FUNCTION_BLOCK IC_KP2_2HB21_IQH3_SF
VAR_INPUT
	pADR_IN:								PVOID;					(* Pointer array input data *)
	cbSIZE_IN:								UDINT;					(* Size array input data *)
	pADR_OUT:								PVOID;					(* Pointer array output data *)
	cbSIZE_OUT:								UDINT;					(* Size array output data *)	
	I_T_Timeout : 							TIME;					// Timeout to check command responses
	I_b_StartRead : 						BOOL;					// Trigger to start read command
	I_b_StartWrite : 						BOOL;					// Trigger to start write command
	I_b_StartSpecialCommand : 				BOOL;					// Trigger to start special command (user defined command)
	I_b_UserMemory_UID : 					BOOL;					//0 := access to User Memory; 1 := access to UID/Fixcode
	I_b_EPC : 								BOOL;					//0 := configuration done by Head1UserMemoryUID active; 1 := access to UII/EPC Code (UHF only)
	I_b_SingleEnhanced : 					BOOL;					// 0 = Single command (one-time) ; 1 = Enhanced command (permanent)
	I_b_Quit : 								BOOL;					// Trigger to start Quit command (abort Enhanced command)
	I_w_StartAddress : 						WORD;					// Startaddress of memory access 
	I_i_WordNumber : 						INT;					// Number of blocks
	I_w_TagType : 							WORD;					// TagType
	I_b_WriteParameter : 					BOOL;					//0 := read access to parameter; 1 := write access to parameter
END_VAR
VAR_OUTPUT
	O_b_Done : 								BOOL;					//0 = tag leave detection zone (Enhanced); 1 = tag access successfully executed
	O_b_NoDataCarrier : 					BOOL;					//0 = tag inside/enter detection zone; 1 = no tag or tag leave detection zone
	O_b_Busy : 								BOOL;					//0 = no command actiive; 1 = command active
	O_b_Finish : 							BOOL;					//0 = command active; 1 = command finished
	O_b_Error : 							BOOL;					//0 = no error state; 1 = error state active; check status value
	O_B_Status : 							BYTE;					//Status value of the command response; error information
	O_B_ReplyCounter : 						BYTE;					//Counter of the command responses; increment each new response
	O_b_EndConfig : 						BOOL;					//1 = parameter access finished
END_VAR
VAR_IN_OUT
	IO_b_SetRestart : 						BOOL;					//Trigger initialisation routine
	IO_b_InitFinish : 						BOOL;					//Initialisation routine finished
	IO_b_StartConfig : 						BOOL;
	UserDataGlobal 	: 						IDENTControl_UserData;	//Data block for read/write data and parameter data
END_VAR
VAR
	IDENTControl_FB_SF		: 				IDENTControl_SF;		//Definition of internal function block for Single Frame Protocol
	SpecialCommand_Internal: 				BOOL;					//internal signal for trigger of Special command
	ConfigActive : 							BOOL;					//execution of Special command active
	StateConfig : 							INT;					//state of the execution list
	Done_Internal : 						BOOL;					//Special command finished
	i : 									INT := 0;				//counter
END_VAR

	(*
	#############################################################################################
	
	General Header
	------------------------------------------------------------------------------------------
	Short description:  Function Block for IC-KP2-2HB21 SingleFrame with Parameter configuration for IQH3-FP-V1
	Version:            1.0
	Name:               IC-KP2-2HB21 Singleframe Protocol with HF Parameter configuration for IQH3-FP-V1
	Date:               2024-10-08
	Company:            Pepperl+Fuchs SE
	Author:             Karsten Reinhardt
	EMail:              kreinhardt@de.pepperl-fuchs.com
	Phone:              +49 (0) 621 776 1736

	Changes 1.0: first release
	    - function block include a further function block for standard read/write command without automatic parameter
	    configuration;    
	    - read and write access for different HF parameter
		- based on function block for IC-KP2-1HB17 TIA Portal Profinet for parameter access of IQH3-FP-V1
	
	------------------------------------------------------------------------------------------
	    
	#############################################################################################
	*)

	(*input SpecialCommand hand over to internal signal*)
	SpecialCommand_Internal                   			:= I_b_StartSpecialCommand;

	(*Increase the state of the configuration counter*)
	IF ConfigActive = TRUE AND O_b_Done = TRUE THEN
	    ConfigActive                         			:= FALSE;
	    StateConfig                          			:= StateConfig + 1;
	END_IF;
	
	(*Set Status of the configuration counter to 1 with the trigger for the start of the configuration*)
	IF IO_b_StartConfig = TRUE THEN
	    StateConfig                          			:= 1;
	    IO_b_StartConfig                          		:= FALSE;
	    O_b_EndConfig                             		:= FALSE;
	END_IF;

	IF NOT ConfigActive THEN
	    CASE StateConfig OF
	            
	        0: (* ***** Idle state ***** *)
	            ;
	            
	        1:  (*Additional Information - Parameter IF; transmit a further information telegram with RSSI value;
	            if this parameter is activated a further status 16#0B telegram will transmitted by the evaluation
	            unit; this telegram follows directly after the status 16#00 telegram which contains the read in data
	            of a tag; the status 16#0B telegram with the information will send only one time after the tag is detected;
	            in default setting the parameter is switched off and no additional information are transmit*)
	            IF I_b_WriteParameter = TRUE THEN
	                UserDataGlobal.SpecialCommand[0] 	:= 16#BF;
	            ELSE
					UserDataGlobal.SpecialCommand[0] 	:= 16#BE;	                
	            END_IF;
	            UserDataGlobal.SpecialCommand[1]        := 16#00;
	            UserDataGlobal.SpecialCommand[2]        := 16#00;
	            UserDataGlobal.SpecialCommand[3]        := 16#51;      //SystemCode Q
	            UserDataGlobal.SpecialCommand[4]        := 16#49;      //Parameter sign High Byte 'I'
	            UserDataGlobal.SpecialCommand[5]        := 16#46;      //Parameter sign Low Byte 'F'
				IF I_b_WriteParameter = TRUE THEN
	                UserDataGlobal.SpecialCommand[6]    := 16#00;    //Length Parameter High Byte 
	                UserDataGlobal.SpecialCommand[7]    := 16#01;    //Length Parameter Low Byte 
	                UserDataGlobal.SpecialCommand[8]    := UserDataGlobal.WriteParam_IF;    //Parameter value; 16#00 Switched off; 16#01 Switched on
	            ELSE
	                UserDataGlobal.SpecialCommand[6]    := 16#00;    //Length Parameter High Byte 
	                UserDataGlobal.SpecialCommand[7]    := 16#00;    //Length Parameter Low Byte 
	                UserDataGlobal.SpecialCommand[8]    := 16#00;
	            END_IF;
	            SpecialCommand_Internal       			:= TRUE;
	            ConfigActive                 			:= TRUE;            
				
	        2:  (*AFI to request - Parameter AF; *)
	            IF I_b_WriteParameter = TRUE THEN
	                UserDataGlobal.SpecialCommand[0]    := 16#BF;
	            ELSE
	                UserDataGlobal.SpecialCommand[0]    := 16#BE;
	            END_IF;
	            UserDataGlobal.SpecialCommand[1]        := 16#00;
	            UserDataGlobal.SpecialCommand[2]        := 16#00;
	            UserDataGlobal.SpecialCommand[3]        := 16#51;      //SystemCode Q
	            UserDataGlobal.SpecialCommand[4]        := 16#41;      //Parameter sign High Byte 'A'
	            UserDataGlobal.SpecialCommand[5]        := 16#46;      //Parameter sign Low Byte 'F'
	            IF I_b_WriteParameter = TRUE THEN
	                UserDataGlobal.SpecialCommand[6]    := 16#00;    //Length Parameter High Byte 
	                UserDataGlobal.SpecialCommand[7]    := 16#01;    //Length Parameter Low Byte 
	                UserDataGlobal.SpecialCommand[8]    := UserDataGlobal.WriteParam_AF;    //Parameter value; 16#00 = all tags; Range between 16#00 and 16#FF
	            ELSE
	                UserDataGlobal.SpecialCommand[6]    := 16#00;    //Length Parameter High Byte 
	                UserDataGlobal.SpecialCommand[7]    := 16#00;    //Length Parameter Low Byte 
	                UserDataGlobal.SpecialCommand[8]    := 16#00;    //Parameter value; 
	            END_IF;
	            SpecialCommand_Internal       			:= TRUE;
	            ConfigActive 							:= TRUE;

	        3:  (*Enhanced Status 5 - Parameter E5; delay the sending of a status 16#05 telegram which signalise that
	            a tag leaves the detection zone; if there is a inhomogeneous reading zone you have areas in which a tag
	            could not identified; in this case the reader generates a status 16#05 telegram that signalize that a tag 
	            could not accessed; these parameter can delay such telegrams that you can avoid a lot of status 16#05 (no read) 
	            telegrams in a inhomogeneous reading zone*)
	            IF I_b_WriteParameter = TRUE THEN
	                UserDataGlobal.SpecialCommand[0]    := 16#BF;
	            ELSE
	                UserDataGlobal.SpecialCommand[0]    := 16#BE;
	            END_IF;
	            UserDataGlobal.SpecialCommand[1]        := 16#00;
	            UserDataGlobal.SpecialCommand[2]        := 16#00;
	            UserDataGlobal.SpecialCommand[3]        := 16#51;      //SystemCode Q
	            UserDataGlobal.SpecialCommand[4]        := 16#45;      //Parameter sign High Byte 'E'
	            UserDataGlobal.SpecialCommand[5]        := 16#35;      //Parameter sign Low Byte '5'
	            IF I_b_WriteParameter = TRUE THEN
	                UserDataGlobal.SpecialCommand[6]    := 16#00;    //Length Parameter High Byte 
	                UserDataGlobal.SpecialCommand[7]    := 16#01;    //Length Parameter Low Byte 
	                UserDataGlobal.SpecialCommand[8]    := UserDataGlobal.WriteParam_E5;    //Parameter value; value Parameter E5
	                UserDataGlobal.SpecialCommand[9]    := 16#00;    //Parameter value; 
	                UserDataGlobal.SpecialCommand[10]   := 16#00;    //Parameter value; 
	                UserDataGlobal.SpecialCommand[11]   := 16#00;    //Parameter value; 
	            ELSE
	                UserDataGlobal.SpecialCommand[6]    := 16#00;    //Length Parameter High Byte 
	                UserDataGlobal.SpecialCommand[7]    := 16#00;    //Length Parameter Low Byte 
	                UserDataGlobal.SpecialCommand[8]    := 16#00;    //Parameter value; 
	                UserDataGlobal.SpecialCommand[9]    := 16#00;    //Parameter value; 
	                UserDataGlobal.SpecialCommand[10]   := 16#00;    //Parameter value; 
	                UserDataGlobal.SpecialCommand[11]   := 16#00;    //Parameter value; 
	            END_IF;
	            SpecialCommand_Internal       			:= TRUE;
	            ConfigActive                 			:= TRUE;

 			4:  (*Number of Tags - Parameter NT; stop criteria to abort the execution of a Single command; this parameter
	            allows the stop of the command execution if one or a defined number of tags are detected; in default setting
	            the parameter has the value 16#FF and the command does not stop before all invetury rounds are executed; if
	            the value 16#01 is defined the command execution of a Single command stops if one tag is detected during an
	            invetury round; if two tags are detected during an inventury round both tags will transmit*)
	            IF I_b_WriteParameter = TRUE THEN
	                UserDataGlobal.SpecialCommand[0]    := 16#BF;
	            ELSE
	                UserDataGlobal.SpecialCommand[0]    := 16#BE;
	            END_IF;
	            UserDataGlobal.SpecialCommand[1]        := 16#00;
	            UserDataGlobal.SpecialCommand[2]        := 16#00;
	            UserDataGlobal.SpecialCommand[3]        := 16#51;      //SystemCode Q
	            UserDataGlobal.SpecialCommand[4]        := 16#4E;      //Parameter sign High Byte 'N'
	            UserDataGlobal.SpecialCommand[5]        := 16#54;      //Parameter sign Low Byte 'T'
	            IF I_b_WriteParameter = TRUE THEN
	                UserDataGlobal.SpecialCommand[6]    := 16#00;    //Length Parameter High Byte 
	                UserDataGlobal.SpecialCommand[7]    := 16#01;    //Length Parameter Low Byte 
	                UserDataGlobal.SpecialCommand[8]    := UserDataGlobal.WriteParam_NT;    //Parameter value; 16#FF = Switched off; Default setting
	            ELSE
	                UserDataGlobal.SpecialCommand[6]    := 16#00;    //Length Parameter High Byte 
	                UserDataGlobal.SpecialCommand[7]    := 16#00;    //Length Parameter Low Byte 
	                UserDataGlobal.SpecialCommand[8]    := 16#00;    //Parameter value;
	            END_IF;
	            SpecialCommand_Internal       			:= TRUE;
	            ConfigActive                 			:= TRUE;

	        5: (*Protocol Mode - Parameter QV; defines the communication protocol of the head; in default setting the
	            head communicates with the SingleFrame protocol; this allows the identification of several tags inside
	            the detection zone; it is possible to switch the protocol to MultiFrame, but than the function block
	            is incompatible*)
	            IF I_b_WriteParameter = TRUE THEN
	                UserDataGlobal.SpecialCommand[0]    := 16#BF;
	            ELSE
	                UserDataGlobal.SpecialCommand[0]    := 16#BE;
	            END_IF;
	            UserDataGlobal.SpecialCommand[1]        := 16#00;
	            UserDataGlobal.SpecialCommand[2]        := 16#00;
	            UserDataGlobal.SpecialCommand[3]        := 16#51;      //SystemCode Q
	            UserDataGlobal.SpecialCommand[4]        := 16#51;      //Parameter sign High Byte 'Q'
	            UserDataGlobal.SpecialCommand[5]        := 16#56;      //Parameter sign Low Byte 'V'
	            IF I_b_WriteParameter = TRUE THEN
	                UserDataGlobal.SpecialCommand[6]    := 16#00;    //Length Parameter High Byte 
	                UserDataGlobal.SpecialCommand[7]    := 16#01;    //Length Parameter Low Byte 
	                UserDataGlobal.SpecialCommand[8]    := UserDataGlobal.WriteParam_QV;    //Parameter value; 
	            ELSE
	                UserDataGlobal.SpecialCommand[6]    := 16#00;    //Length Parameter High Byte 
	                UserDataGlobal.SpecialCommand[7]    := 16#00;    //Length Parameter Low Byte 
	                UserDataGlobal.SpecialCommand[8]    := 16#00;    //Parameter value; 
	            END_IF;
	            SpecialCommand_Internal       			:= TRUE;
	            ConfigActive                 			:= TRUE;
	            
	        6:  (*Q Value - Parameter QW; defines the number of time slots on the air interface with 2^Q; the number of
	            time slots should be fit to the number of tags which should be identified*)
	            IF I_b_WriteParameter = TRUE THEN
	                UserDataGlobal.SpecialCommand[0]    := 16#BF;
	            ELSE
	                UserDataGlobal.SpecialCommand[0]    := 16#BE;
	            END_IF;
	            UserDataGlobal.SpecialCommand[1]        := 16#00;
	            UserDataGlobal.SpecialCommand[2]        := 16#00;
	            UserDataGlobal.SpecialCommand[3]        := 16#51;      //SystemCode Q
	            UserDataGlobal.SpecialCommand[4]        := 16#51;      //Parameter sign High Byte 'Q'
	            UserDataGlobal.SpecialCommand[5]        := 16#57;      //Parameter sign Low Byte 'W'
	            IF I_b_WriteParameter = TRUE THEN
	                UserDataGlobal.SpecialCommand[6]    := 16#00;    //Length Parameter High Byte 
	                UserDataGlobal.SpecialCommand[7]    := 16#01;    //Length Parameter Low Byte 
	                UserDataGlobal.SpecialCommand[8]    := UserDataGlobal.WriteParam_QW;    //Parameter value; 
	            ELSE
	                UserDataGlobal.SpecialCommand[6]    := 16#00;    //Length Parameter High Byte 
	                UserDataGlobal.SpecialCommand[7]    := 16#00;    //Length Parameter Low Byte 
	                UserDataGlobal.SpecialCommand[8]    := 16#00;    //Parameter value; 
	            END_IF;
	            SpecialCommand_Internal       			:= TRUE;
	            ConfigActive                 			:= TRUE;
	            
	        7:  (*Tries allowed - Parameter TA; defines the number of allowed tries for the identification of a tag*)
	            IF I_b_WriteParameter = TRUE THEN
	                UserDataGlobal.SpecialCommand[0]    := 16#BF;
	            ELSE
	                UserDataGlobal.SpecialCommand[0]    := 16#BE;
	            END_IF;
	            UserDataGlobal.SpecialCommand[1]        := 16#00;
	            UserDataGlobal.SpecialCommand[2]        := 16#00;
	            UserDataGlobal.SpecialCommand[3]        := 16#51;      //SystemCode Q
	            UserDataGlobal.SpecialCommand[4]        := 16#54;      //Parameter sign High Byte 'T'
	            UserDataGlobal.SpecialCommand[5]        := 16#41;      //Parameter sign Low Byte 'A'
	            IF I_b_WriteParameter = TRUE THEN
	                UserDataGlobal.SpecialCommand[6]    := 16#00;    //Length Parameter High Byte 
	                UserDataGlobal.SpecialCommand[7]    := 16#01;    //Length Parameter Low Byte 
	                UserDataGlobal.SpecialCommand[8]    := UserDataGlobal.WriteParam_TA;    //Parameter value; 
	            ELSE
	                UserDataGlobal.SpecialCommand[6]    := 16#00;    //Length Parameter High Byte 
	                UserDataGlobal.SpecialCommand[7]    := 16#00;    //Length Parameter Low Byte 
	                UserDataGlobal.SpecialCommand[8]    := 16#00;    //Parameter value; 
	            END_IF;
	            SpecialCommand_Internal       			:= TRUE;
	            ConfigActive                 			:= TRUE;

			8:  (*Power Transmit - Parameter PT; defines the output power of the RFID antenna; value between 16#0001 up tp 16#0004
	            16#0001 = Min; 16#0002 = Eco; 16#0003 = Normal; 16#0004 = Max Power*)
	            IF I_b_WriteParameter = TRUE THEN
	                UserDataGlobal.SpecialCommand[0]    := 16#BF;
	            ELSE
	                UserDataGlobal.SpecialCommand[0]    := 16#BE;
	            END_IF;
	            UserDataGlobal.SpecialCommand[1]        := 16#00;
	            UserDataGlobal.SpecialCommand[2]        := 16#00;
	            UserDataGlobal.SpecialCommand[3]        := 16#51;      //SystemCode Q
	            UserDataGlobal.SpecialCommand[4]        := 16#50;      //Parameter sign High Byte 'P'
	            UserDataGlobal.SpecialCommand[5]        := 16#54;      //Parameter sign Low Byte 'T'
	            IF I_b_WriteParameter = TRUE THEN
	                UserDataGlobal.SpecialCommand[6]    := 16#00;    //Length Parameter High Byte 
	                UserDataGlobal.SpecialCommand[7]    := 16#02;    //Length Parameter Low Byte 
	                UserDataGlobal.SpecialCommand[8]    := WORD_TO_BYTE( SHL(UserDataGlobal.WriteParam_PT, 8));
	                UserDataGlobal.SpecialCommand[9]    := WORD_TO_BYTE(UserDataGlobal.WriteParam_PT);
	            ELSE
	                UserDataGlobal.SpecialCommand[6]    := 16#00;    //Length Parameter High Byte 
	                UserDataGlobal.SpecialCommand[7]    := 16#00;    //Length Parameter Low Byte 
	                UserDataGlobal.SpecialCommand[8]    := 16#00;    //Parameter value; 
	                UserDataGlobal.SpecialCommand[9]    := 16#00;    //Parameter value; 
	            END_IF;
	            SpecialCommand_Internal       			:= TRUE;
	            ConfigActive                 			:= TRUE;
				
			9:  (*Data Rate - Parameter DR; Data Rate for read operation; Default is 16#00 = normal; fast read mode = 16#01; valid for IQC21/33/34/37/39/50 *)
	            IF I_b_WriteParameter = TRUE THEN
	                UserDataGlobal.SpecialCommand[0]    := 16#BF;
	            ELSE
	                UserDataGlobal.SpecialCommand[0]    := 16#BE;
	            END_IF;
	            UserDataGlobal.SpecialCommand[1]        := 16#00;
	            UserDataGlobal.SpecialCommand[2]        := 16#00;
	            UserDataGlobal.SpecialCommand[3]        := 16#51;      //SystemCode Q
	            UserDataGlobal.SpecialCommand[4]        := 16#44;      //Parameter sign High Byte 'D'
	            UserDataGlobal.SpecialCommand[5]        := 16#52;      //Parameter sign Low Byte 'R'
	            IF I_b_WriteParameter = TRUE THEN
	                UserDataGlobal.SpecialCommand[6]    := 16#00;    //Length Parameter High Byte 
	                UserDataGlobal.SpecialCommand[7]    := 16#01;    //Length Parameter Low Byte 
	                UserDataGlobal.SpecialCommand[8]    := UserDataGlobal.WriteParam_DR;    //Parameter value; 
	                UserDataGlobal.SpecialCommand[9]    := 16#00;    //Parameter value; 
	            ELSE
	                UserDataGlobal.SpecialCommand[6]    := 16#00;    //Length Parameter High Byte 
	                UserDataGlobal.SpecialCommand[7]    := 16#00;    //Length Parameter Low Byte 
	                UserDataGlobal.SpecialCommand[8]    := 16#00;    //Parameter value; 
	                UserDataGlobal.SpecialCommand[9]    := 16#00;    //Parameter value; 
	            END_IF;
	            SpecialCommand_Internal       			:= TRUE;
	            ConfigActive                 			:= TRUE;
				
	        10:  (*Tag ID filterung on UID - Parameter TI; leading part of the UID*)
	            IF I_b_WriteParameter = TRUE THEN
	                UserDataGlobal.SpecialCommand[0]    := 16#BF;
	            ELSE
	                UserDataGlobal.SpecialCommand[0]    := 16#BE;
	            END_IF;
	            UserDataGlobal.SpecialCommand[1]        := 16#00;
	            UserDataGlobal.SpecialCommand[2]        := 16#00;
	            UserDataGlobal.SpecialCommand[3]        := 16#51;      //SystemCode Q
	            UserDataGlobal.SpecialCommand[4]        := 16#54;      //Parameter sign High Byte 'T'
	            UserDataGlobal.SpecialCommand[5]        := 16#49;      //Parameter sign Low Byte 'I'
	            IF I_b_WriteParameter = TRUE THEN
	                UserDataGlobal.SpecialCommand[6]    := UserDataGlobal.WriteParam_TI[0];    //Length Parameter High Byte 
	                UserDataGlobal.SpecialCommand[7]    := UserDataGlobal.WriteParam_TI[1];    //Length Parameter Low Byte 
	                UserDataGlobal.SpecialCommand[8]    := UserDataGlobal.WriteParam_TI[2];   //Parameter value; 
	                UserDataGlobal.SpecialCommand[9]    := UserDataGlobal.WriteParam_TI[3];   //Parameter value;
	                UserDataGlobal.SpecialCommand[10]   := UserDataGlobal.WriteParam_TI[4];   //Parameter value;
	                UserDataGlobal.SpecialCommand[11]   := UserDataGlobal.WriteParam_TI[5];    //Parameter value;
	                UserDataGlobal.SpecialCommand[12]   := UserDataGlobal.WriteParam_TI[6];    //Parameter value;
	                UserDataGlobal.SpecialCommand[13]   := UserDataGlobal.WriteParam_TI[7];    //Parameter value;
	                UserDataGlobal.SpecialCommand[14]   := UserDataGlobal.WriteParam_TI[8];   //Parameter value;
	                UserDataGlobal.SpecialCommand[15]   := UserDataGlobal.WriteParam_TI[9];   //Parameter value;
	            ELSE
	                UserDataGlobal.SpecialCommand[6]    := 16#00;    //Length Parameter High Byte 
	                UserDataGlobal.SpecialCommand[7]    := 16#00;    //Length Parameter Low Byte 
	                UserDataGlobal.SpecialCommand[8]    := 16#00;    //Parameter value; 
	            END_IF;
	            SpecialCommand_Internal       			:= TRUE;
	            ConfigActive                 			:= TRUE;				
				
	        11:  (*Over temperature handling - Parameter TO; defines the behavior if over temperature occures;
	              16#00 = Switch off; 16#01 = reduce power; 16#02 = reduce duty cycle*)
	            IF I_b_WriteParameter = TRUE THEN
	                UserDataGlobal.SpecialCommand[0]    := 16#BF;
	            ELSE
	                UserDataGlobal.SpecialCommand[0]    := 16#BE;
	            END_IF;
	            UserDataGlobal.SpecialCommand[1]        := 16#00;
	            UserDataGlobal.SpecialCommand[2]        := 16#00;
	            UserDataGlobal.SpecialCommand[3]        := 16#51;      //SystemCode Q
	            UserDataGlobal.SpecialCommand[4]        := 16#54;      //Parameter sign High Byte 'T'
	            UserDataGlobal.SpecialCommand[5]        := 16#4F;      //Parameter sign Low Byte 'O'
	            IF I_b_WriteParameter = TRUE THEN
	                UserDataGlobal.SpecialCommand[6]    := 16#00;    //Length Parameter High Byte 
	                UserDataGlobal.SpecialCommand[7]    := 16#01;    //Length Parameter Low Byte 
	                UserDataGlobal.SpecialCommand[8]    := UserDataGlobal.WriteParam_TO;    //Parameter value; 
	                UserDataGlobal.SpecialCommand[9]    := 16#00;    //Parameter value; 
	            ELSE
	                UserDataGlobal.SpecialCommand[6]    := 16#00;    //Length Parameter High Byte 
	                UserDataGlobal.SpecialCommand[7]    := 16#00;    //Length Parameter Low Byte 
	                UserDataGlobal.SpecialCommand[8]    := 16#00;    //Parameter value; 
	                UserDataGlobal.SpecialCommand[9]    := 16#00;    //Parameter value; 
	            END_IF;
	            SpecialCommand_Internal 				:= TRUE;
	            ConfigActive 							:= TRUE;

	        12:    (*TagType (change Tag) - Parameter CT; read out the configured Tag type which was configured by the Change Tag command
	                during initialisation routine*)
	            UserDataGlobal.SpecialCommand[0]        := 16#BE;
	            UserDataGlobal.SpecialCommand[1]        := 16#00;
	            UserDataGlobal.SpecialCommand[2]        := 16#00;
	            UserDataGlobal.SpecialCommand[3]        := 16#51;      //SystemCode Q
	            UserDataGlobal.SpecialCommand[4]        := 16#43;      //Parameter sign High Byte 'C'
	            UserDataGlobal.SpecialCommand[5]        := 16#54;      //Parameter sign Low Byte 'T'
	            UserDataGlobal.SpecialCommand[6]        := 16#00;    //Length Parameter High Byte 
	            UserDataGlobal.SpecialCommand[7]        := 16#00;    //Length Parameter Low Byte 
	            UserDataGlobal.SpecialCommand[8]        := 16#00;    //Parameter value; 
	            
	            SpecialCommand_Internal       			:= TRUE;
	            ConfigActive                 			:= TRUE;				
				
	        13: (*Operating hours - Parameter OH; read out the hours the head was operating*)
	            UserDataGlobal.SpecialCommand[0]        := 16#BE;
	            UserDataGlobal.SpecialCommand[1]        := 16#00;
	            UserDataGlobal.SpecialCommand[2]        := 16#00;
	            UserDataGlobal.SpecialCommand[3]        := 16#51;      //SystemCode Q
	            UserDataGlobal.SpecialCommand[4]        := 16#4F;      //Parameter sign High Byte 'O'
	            UserDataGlobal.SpecialCommand[5]        := 16#48;      //Parameter sign Low Byte 'H'
	            UserDataGlobal.SpecialCommand[6]        := 16#00;    //Length Parameter High Byte 
	            UserDataGlobal.SpecialCommand[7]        := 16#00;    //Length Parameter Low Byte 
	            UserDataGlobal.SpecialCommand[8]        := 16#00;    //Parameter value; 
	            
	            SpecialCommand_Internal       			:= TRUE;
	            ConfigActive                 			:= TRUE;				
			
	        14: (*Read Temperatures - Parameter TE; read out the internal device temperature *)
	            UserDataGlobal.SpecialCommand[0]        := 16#BE;
	            UserDataGlobal.SpecialCommand[1]        := 16#00;
	            UserDataGlobal.SpecialCommand[2]        := 16#00;
	            UserDataGlobal.SpecialCommand[3]        := 16#51;      //SystemCode Q
	            UserDataGlobal.SpecialCommand[4]        := 16#54;      //Parameter sign High Byte 'T'
	            UserDataGlobal.SpecialCommand[5]        := 16#45;      //Parameter sign Low Byte 'E'
	            UserDataGlobal.SpecialCommand[6]        := 16#00;    //Length Parameter High Byte 
	            UserDataGlobal.SpecialCommand[7]        := 16#00;    //Length Parameter Low Byte 
	            UserDataGlobal.SpecialCommand[8]        := 16#00;    //Parameter value; 
	            
	            SpecialCommand_Internal       			:= TRUE;
	            ConfigActive                 			:= TRUE;				

	        15:  (*Read Voltages - Parameter VO; read out internal voltages*)
	            UserDataGlobal.SpecialCommand[0]        := 16#BE;
	            UserDataGlobal.SpecialCommand[1]        := 16#00;
	            UserDataGlobal.SpecialCommand[2]        := 16#00;
	            UserDataGlobal.SpecialCommand[3]        := 16#51;      //SystemCode Q
	            UserDataGlobal.SpecialCommand[4]        := 16#56;      //Parameter sign High Byte 'V'
	            UserDataGlobal.SpecialCommand[5]        := 16#4F;      //Parameter sign Low Byte 'O'
	            UserDataGlobal.SpecialCommand[6]        := 16#00;    //Length Parameter High Byte 
	            UserDataGlobal.SpecialCommand[7]        := 16#00;    //Length Parameter Low Byte 
	            UserDataGlobal.SpecialCommand[8]        := 16#00;    //Parameter value; 
	            
	            SpecialCommand_Internal       			:= TRUE;
	            ConfigActive                 			:= TRUE;

			16:  (*Sequence Mode - Parameter FR; internal parameter do not change*)
	            IF I_b_WriteParameter = TRUE THEN
	                UserDataGlobal.SpecialCommand[0]    := 16#BF;
	            ELSE
	                UserDataGlobal.SpecialCommand[0]    := 16#BE;
	            END_IF;
	            UserDataGlobal.SpecialCommand[1]        := 16#00;
	            UserDataGlobal.SpecialCommand[2]        := 16#00;
	            UserDataGlobal.SpecialCommand[3]        := 16#51;      //SystemCode Q
	            UserDataGlobal.SpecialCommand[4]        := 16#46;      //Parameter sign High Byte 'F'
	            UserDataGlobal.SpecialCommand[5]        := 16#52;      //Parameter sign Low Byte 'R'
	            IF I_b_WriteParameter = TRUE THEN
	                UserDataGlobal.SpecialCommand[6]    := 16#00;    //Length Parameter High Byte 
	                UserDataGlobal.SpecialCommand[7]    := 16#01;    //Length Parameter Low Byte 
	                UserDataGlobal.SpecialCommand[8]    := UserDataGlobal.WriteParam_FR;    //Parameter value; 
	                UserDataGlobal.SpecialCommand[9]    := 16#00;    //Parameter value; 
	            ELSE
	                UserDataGlobal.SpecialCommand[6]    := 16#00;    //Length Parameter High Byte 
	                UserDataGlobal.SpecialCommand[7]    := 16#00;    //Length Parameter Low Byte 
	                UserDataGlobal.SpecialCommand[8]    := 16#00;    //Parameter value; 
	                UserDataGlobal.SpecialCommand[9]    := 16#00;    //Parameter value; 
	            END_IF;
	            SpecialCommand_Internal       			:= TRUE;
	            ConfigActive                 			:= TRUE;
				
	        17:  (*Read Version GIT - Parameter RV; internal parameter*)
	            UserDataGlobal.SpecialCommand[0]        := 16#BE;
	            UserDataGlobal.SpecialCommand[1]        := 16#00;
	            UserDataGlobal.SpecialCommand[2]        := 16#00;
	            UserDataGlobal.SpecialCommand[3]        := 16#51;      //SystemCode Q
	            UserDataGlobal.SpecialCommand[4]        := 16#52;      //Parameter sign High Byte 'R'
	            UserDataGlobal.SpecialCommand[5]        := 16#56;      //Parameter sign Low Byte 'V'
	            UserDataGlobal.SpecialCommand[6]        := 16#00;    //Length Parameter High Byte 
	            UserDataGlobal.SpecialCommand[7]        := 16#00;    //Length Parameter Low Byte 
	            UserDataGlobal.SpecialCommand[8]        := 16#00;    //Parameter value; 16#02 --> Filter 2
	            
	            SpecialCommand_Internal       			:= TRUE;
	            ConfigActive                 			:= TRUE;				

	        18:  (*Serial Number - Parameter SN; Read out serial number STM32 IC; internal parameter*)
	            UserDataGlobal.SpecialCommand[0]        := 16#BE;
	            UserDataGlobal.SpecialCommand[1]        := 16#00;
	            UserDataGlobal.SpecialCommand[2]        := 16#00;
	            UserDataGlobal.SpecialCommand[3]        := 16#51;      //SystemCode Q
	            UserDataGlobal.SpecialCommand[4]        := 16#53;      //Parameter sign High Byte 'S'
	            UserDataGlobal.SpecialCommand[5]        := 16#4E;      //Parameter sign Low Byte 'N'
	            UserDataGlobal.SpecialCommand[6]        := 16#00;    //Length Parameter High Byte 
	            UserDataGlobal.SpecialCommand[7]        := 16#00;    //Length Parameter Low Byte 
	            UserDataGlobal.SpecialCommand[8]        := 16#00;    //Parameter value; 
	            
	            SpecialCommand_Internal       			:= TRUE;
	            ConfigActive                 			:= TRUE;

	        19:  (*Multiplex Mode - Parameter MM; Read out configuration of MM; internal parameter*)
	            UserDataGlobal.SpecialCommand[0]        := 16#BE;
	            UserDataGlobal.SpecialCommand[1]        := 16#00;
	            UserDataGlobal.SpecialCommand[2]        := 16#00;
	            UserDataGlobal.SpecialCommand[3]        := 16#51;      //SystemCode Q
	            UserDataGlobal.SpecialCommand[4]        := 16#4D;      //Parameter sign High Byte 'M'
	            UserDataGlobal.SpecialCommand[5]        := 16#4D;      //Parameter sign Low Byte 'M'
	            UserDataGlobal.SpecialCommand[6]        := 16#00;    //Length Parameter High Byte 
	            UserDataGlobal.SpecialCommand[7]        := 16#00;    //Length Parameter Low Byte 
	            UserDataGlobal.SpecialCommand[8]        := 16#00;    //Parameter value; 
	            
	            SpecialCommand_Internal       			:= TRUE;
	            ConfigActive                 			:= TRUE;
	            
	        20: (*Parameter ST - Status of the front end*)
	            UserDataGlobal.SpecialCommand[0] 		:= 16#BE;
	            UserDataGlobal.SpecialCommand[1] 		:= 16#00;
	            UserDataGlobal.SpecialCommand[2] 		:= 16#00;
	            UserDataGlobal.SpecialCommand[3] 		:= 16#51;      //SystemCode Q
	            UserDataGlobal.SpecialCommand[4] 		:= 16#53;      //Parameter sign High Byte 'S'
	            UserDataGlobal.SpecialCommand[5] 		:= 16#54;      //Parameter sign Low Byte 'T'
	            UserDataGlobal.SpecialCommand[6] 		:= 16#00;    //Length Parameter High Byte 
	            UserDataGlobal.SpecialCommand[7] 		:= 16#00;    //Length Parameter Low Byte 
	           	UserDataGlobal.SpecialCommand[8] 		:= 16#00;    //Parameter value; 
	            
	            SpecialCommand_Internal 				:= TRUE;
	            ConfigActive 							:= TRUE;				
								
	        21:
	            StateConfig                  			:= 0; (* Go to idle state *)
	            
	    END_CASE;
	END_IF;	

IDENTControl_FB_SF(
	pADR_IN	:= pADR_IN,									(* Pointer array input data *)
	cbSIZE_IN := cbSIZE_IN,								(* Size array input data *)
	pADR_OUT := pADR_OUT,								(* Pointer array output data *)
	cbSIZE_OUT := cbSIZE_OUT,							(* Size array output data *)
	I_T_Timeout := I_T_Timeout, 						// Timeout to check command responses
	I_b_StartRead := I_b_StartRead, 					// Trigger to start read command
	I_b_StartWrite := I_b_StartWrite, 					// Trigger to start write command
	I_b_StartSpecialCommand	:= SpecialCommand_Internal, // Trigger to start special command (user defined command)
	I_b_UserMemory_UID := I_b_UserMemory_UID, 			//0 := access to User Memory; 1 := access to UID/Fixcode
	I_b_EPC := I_b_EPC,									//0 := configuration done by Head1UserMemoryUID active; 1 := access to UII/EPC Code (UHF only)
	I_b_SingleEnhanced := I_b_SingleEnhanced , 			// 0 = Single command (one-time) ; 1 = Enhanced command (permanent)
	I_b_Quit := I_b_Quit, 								// Trigger to start Quit command (abort Enhanced command)
	I_w_StartAddress := I_w_StartAddress, 				// Startaddress of memory access 
	I_i_WordNumber := I_i_WordNumber,					// Number of blocks 
	I_w_TagType := I_w_TagType, 						// TagType
	O_b_Done => Done_Internal, 							//0 = tag leave detection zone (Enhanced); 1 = tag access successfully executed
	O_b_NoDataCarrier => O_b_NoDataCarrier, 			//0 = tag inside/enter detection zone; 1 = no tag or tag leave detection zone
	O_b_Busy => O_b_Busy, 								//0 = no command actiive; 1 = command active
	O_b_Finish => O_b_Finish, 							//0 = command active; 1 = command finished
	O_b_Error => O_b_Error, 							//0 = no error state; 1 = error state active; check status value
	O_B_Status => O_B_Status, 							//Status value of the command response; error information
	O_B_ReplyCounter => O_B_ReplyCounter,				//Counter of the command responses; increment each new response
	IO_b_SetRestart := IO_b_SetRestart, 				//Trigger initialisation routine
	IO_b_InitFinish := IO_b_InitFinish,					//Initialisation routine finished
	UserData := UserDataGlobal							//Data block for read/write data
	);

	
	(*Copy read in information from parameter IF*)
	IF StateConfig = 1 AND Done_Internal = TRUE THEN
	    UserDataGlobal.ReadParam_IF               		:= UserDataGlobal.ReadData[0];
	END_IF;
	(*Copy read in information from parameter AF*)
	IF StateConfig = 2 AND Done_Internal = TRUE THEN
	    UserDataGlobal.ReadParam_AF               		:= UserDataGlobal.ReadData[0];
	END_IF;
	(*Copy read in information from parameter E5*)
	IF StateConfig = 3 AND Done_Internal = TRUE THEN
	    UserDataGlobal.ReadParam_E5               		:= UserDataGlobal.ReadData[0];
	END_IF;
	(*Copy read in information from parameter NT*)
	IF StateConfig = 4 AND Done_Internal = TRUE THEN
	    UserDataGlobal.ReadParam_NT               		:= UserDataGlobal.ReadData[0];
	END_IF;	
	(*Copy read in information from parameter QV*)
	IF StateConfig = 5 AND Done_Internal = TRUE THEN
		UserDataGlobal.ReadParam_QV 					:= UserDataGlobal.ReadData[0];
	END_IF;
	(*Copy read in information from parameter QW*)
	IF StateConfig = 6 AND Done_Internal = TRUE THEN
	    UserDataGlobal.ReadParam_QW               		:= UserDataGlobal.ReadData[0];
	END_IF;
	(*Copy read in information from parameter TA*)
	IF StateConfig = 7 AND Done_Internal = TRUE THEN
	    UserDataGlobal.ReadParam_TA               		:= UserDataGlobal.ReadData[0];
	END_IF;
	(*Copy read in information from parameter PT*)
	IF StateConfig = 8 AND Done_internal = TRUE THEN
	    UserDataGlobal.ReadParam_PT 					:= SHL (BYTE_TO_WORD(UserDataGlobal.ReadData[0]), 8) OR UserDataGlobal.ReadData[1];
	END_IF;	
	(*Copy read in information from parameter DR*)
	IF StateConfig = 9 AND Done_internal = TRUE THEN
	    UserDataGlobal.ReadParam_DR               		:= UserDataGlobal.ReadData[0];
	END_IF;	
	(*Copy read in information from parameter TI*)
	IF StateConfig = 10 AND Done_internal = TRUE THEN
	    UserDataGlobal.ReadParam_TI[0]   				:= UserDataGlobal.ReadData[0];
	    UserDataGlobal.ReadParam_TI[1]   				:= UserDataGlobal.ReadData[1];
	    UserDataGlobal.ReadParam_TI[2]   				:= UserDataGlobal.ReadData[2];
	    UserDataGlobal.ReadParam_TI[3]   				:= UserDataGlobal.ReadData[3];
	    UserDataGlobal.ReadParam_TI[4]   				:= UserDataGlobal.ReadData[4];
	    UserDataGlobal.ReadParam_TI[5]   				:= UserDataGlobal.ReadData[5];
	    UserDataGlobal.ReadParam_TI[6]   				:= UserDataGlobal.ReadData[6];
	    UserDataGlobal.ReadParam_TI[7]   				:= UserDataGlobal.ReadData[7];
		UserDataGlobal.ReadParam_TI[8]   				:= UserDataGlobal.ReadData[8];
	    UserDataGlobal.ReadParam_TI[9]   				:= UserDataGlobal.ReadData[9];
	END_IF;
	(*Copy read in information from parameter TO*)
	IF StateConfig = 11 AND Done_internal = TRUE THEN
	    UserDataGlobal.ReadParam_TO               		:= UserDataGlobal.ReadData[0];
	END_IF;		
	(*Copy read in information from parameter CT*)
	IF StateConfig = 12 AND Done_internal = TRUE THEN
	    UserDataGlobal.ReadParam_CT               		:= BYTE_TO_INT(UserDataGlobal.ReadData[0]);
	END_IF;	
	(*Copy read in information from parameter OH*)
	IF StateConfig = 13 AND Done_internal = TRUE THEN
	 	UserDataGlobal.ReadParam_OH[0]            		:= SHL (BYTE_TO_DWORD(UserDataGlobal.ReadData[0]), 24) OR 
														SHL (BYTE_TO_DWORD(UserDataGlobal.ReadData[1]), 16) OR 
														SHL (BYTE_TO_DWORD(UserDataGlobal.ReadData[2]), 8) OR 
														BYTE_TO_DWORD(UserDataGlobal.ReadData[3]); 
 	    UserDataGlobal.ReadParam_OH[1]            		:= SHL (BYTE_TO_DWORD(UserDataGlobal.ReadData[4]), 24) OR 
														SHL (BYTE_TO_DWORD(UserDataGlobal.ReadData[5]), 16) OR 
														SHL (BYTE_TO_DWORD(UserDataGlobal.ReadData[6]), 8) OR 
														BYTE_TO_DWORD(UserDataGlobal.ReadData[7]); 
		UserDataGlobal.ReadParam_OH[2] 					:= UserDataGlobal.ReadParam_OH[0] / 24;
		UserDataGlobal.ReadParam_OH[3] 					:= UserDataGlobal.ReadParam_OH[1] / 24;
		UserDataGlobal.ReadParam_OH[4] 					:= UserDataGlobal.ReadParam_OH[0] / 168;
		UserDataGlobal.ReadParam_OH[5] 					:= UserDataGlobal.ReadParam_OH[1] / 168;
	 END_IF;
	(*Copy read in information from parameter TE*)
	IF StateConfig = 14 AND Done_internal = TRUE THEN
	    UserDataGlobal.ReadParam_TE[0]            		:= BYTE_TO_INT(UserDataGlobal.ReadData[0]);
	    UserDataGlobal.ReadParam_TE[1]            		:= BYTE_TO_INT(UserDataGlobal.ReadData[1]);
	END_IF;	
	(*Copy read in information from parameter VO*)
	IF StateConfig = 15 AND Done_internal = TRUE THEN
	    UserDataGlobal.ReadParam_VO[0]            		:= SHL (BYTE_TO_UINT(UserDataGlobal.ReadData[0]), 8) OR BYTE_TO_UINT (UserDataGlobal.ReadData[1]);
		UserDataGlobal.ReadParam_VO[1]            		:= SHL (BYTE_TO_UINT(UserDataGlobal.ReadData[2]), 8) OR BYTE_TO_UINT (UserDataGlobal.ReadData[3]);
		UserDataGlobal.ReadParam_VO[2]            		:= SHL (BYTE_TO_UINT(UserDataGlobal.ReadData[4]), 8) OR BYTE_TO_UINT (UserDataGlobal.ReadData[5]);
		UserDataGlobal.ReadParam_VO[3]            		:= SHL (BYTE_TO_UINT(UserDataGlobal.ReadData[6]), 8) OR BYTE_TO_UINT (UserDataGlobal.ReadData[7]);
		UserDataGlobal.ReadParam_VO[4]            		:= SHL (BYTE_TO_UINT(UserDataGlobal.ReadData[8]), 8) OR BYTE_TO_UINT (UserDataGlobal.ReadData[9]);
		UserDataGlobal.ReadParam_VO[5]            		:= SHL (BYTE_TO_UINT(UserDataGlobal.ReadData[10]), 8) OR BYTE_TO_UINT (UserDataGlobal.ReadData[11]);
		UserDataGlobal.ReadParam_VO[6]            		:= SHL (BYTE_TO_UINT(UserDataGlobal.ReadData[12]), 8) OR BYTE_TO_UINT (UserDataGlobal.ReadData[13]);
		UserDataGlobal.ReadParam_VO[7]            		:= SHL (BYTE_TO_UINT(UserDataGlobal.ReadData[14]), 8) OR BYTE_TO_UINT (UserDataGlobal.ReadData[15]);
		UserDataGlobal.ReadParam_VO[8]            		:= SHL (BYTE_TO_UINT(UserDataGlobal.ReadData[16]), 8) OR BYTE_TO_UINT (UserDataGlobal.ReadData[17]);
		UserDataGlobal.ReadParam_VO[9]            		:= SHL (BYTE_TO_UINT(UserDataGlobal.ReadData[18]), 8) OR BYTE_TO_UINT (UserDataGlobal.ReadData[19]);			    
	END_IF;
	(*Copy read in information from parameter FR*)
	IF StateConfig = 16 AND Done_internal = TRUE THEN
	    UserDataGlobal.ReadParam_FR               		:= UserDataGlobal.ReadData[0];
	END_IF;
	(*Copy read in information from parameter RV*)
	IF StateConfig = 17 AND Done_internal = TRUE THEN
	    FOR i := 0 TO 55 BY 1 DO
		UserDataGlobal.ReadParam_RV[i]            		:= UserDataGlobal.ReadData[i];	
		END_FOR;
	END_IF;
	(*Copy read in information from parameter SN*)
	IF StateConfig = 18 AND Done_internal = TRUE THEN
		FOR i := 0 TO 11 BY 1 DO
		UserDataGlobal.ReadParam_SN[i]            		:= UserDataGlobal.ReadData[i];	
		END_FOR;
	END_IF;	
(*Copy read in information from parameter MM*)
	IF StateConfig = 19 AND Done_internal = TRUE THEN
	    UserDataGlobal.ReadParam_MM               		:= UserDataGlobal.ReadData[0];
	END_IF;
	(*Copy read in information from parameter ST*)
	IF StateConfig = 20 AND Done_internal = TRUE THEN
	    UserDataGlobal.ReadParam_ST[0]					:= UserDataGlobal.ReadData[0];
	    UserDataGlobal.ReadParam_ST[1]					:= UserDataGlobal.ReadData[1];
	END_IF;		
	
	IF StateConfig = 20 AND Done_Internal = TRUE THEN
	    O_b_EndConfig 									:= TRUE;
	END_IF;
	
	O_b_Done                                      		:= Done_internal;
	
	IF SpecialCommand_Internal = TRUE THEN
	    SpecialCommand_Internal                  		:= FALSE;
	END_IF;

END_FUNCTION_BLOCK
